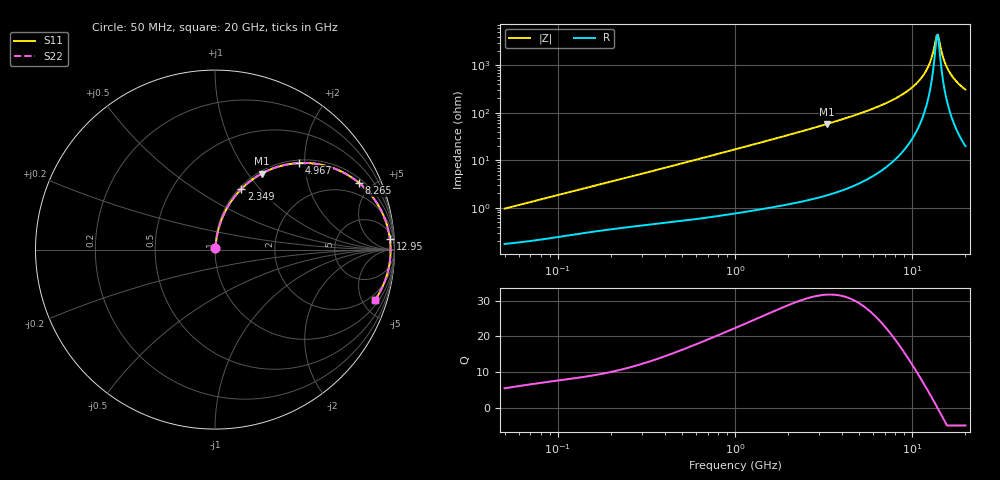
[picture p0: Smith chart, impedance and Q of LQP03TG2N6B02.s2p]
!Murata Part Number: LQP03TG2N6B02
!These Parameters are Measured in Series Mode Connection
!  o--[Z]--o
!Port1  Port2
!  o-------o
!Freq. Start=50[MHz] Stop=20[GHz], 401[Steps]
# Hz S RI R 50
!Freq.(Hz) S11(Real) S11(Imag) S21(Real) S21(Imag) S12(Real) S12(Imag) S22(Real) S22(Imag)
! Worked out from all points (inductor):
!   401 points, 50 MHz to 20 GHz, reference 50 ohm
!   read as one part in series: L = 2.98 nH near 51.52 MHz
!   highest Q = 31.7 at 3.314 GHz (marker M1), where L = 2.79 nH
!   self-resonance near 13.75 GHz
!   S11 on the Smith chart (normalised r, x): 50 MHz: 1.00, +0.02; 2.349 GHz: 1.03, +0.80; 4.967 GHz: 1.06, +1.88; 8.265 GHz: 1.23, +4.21; 12.95 GHz: 12, +29; 20 GHz: 1.40, -6.13
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5e7  0.00182 0.0094  0.9982 -0.0094  0.9982 -0.0094  0.00182 0.0094
1.364002e8  0.00348 0.0245  0.9965 -0.0245  0.9965 -0.0245  0.00348 0.0245
3.721004e8  0.00867 0.0634  0.9913 -0.0634  0.9913 -0.0634  0.00867 0.0634
1e9  0.0348 0.1621  0.9652 -0.1621  0.9652 -0.1621  0.0348 0.1621
2.348516e9  0.147 0.3379  0.853 -0.3379  0.853 -0.3379  0.147 0.3379
2.728004e9  0.189 0.3758  0.811 -0.3758  0.811 -0.3758  0.189 0.3758
3.314454e9  0.2595 0.4229  0.7405 -0.4229  0.7405 -0.4229  0.2595 0.4229
4.966507e9  0.4702 0.4824  0.5298 -0.4824  0.5298 -0.4824  0.4702 0.4824
7.442007e9  0.7376 0.417  0.2624 -0.417  0.2624 -0.417  0.7376 0.417
8.264682e9  0.8032 0.3711  0.1968 -0.3711  0.1968 -0.3711  0.8032 0.3711
9.745021e9  0.8913 0.2752  0.1087 -0.2752  0.1087 -0.2752  0.8913 0.2752
1.098561e10  0.9387 0.1899  0.0613 -0.1899  0.0613 -0.1899  0.9387 0.1899
1.201863e10  0.9628 0.1197  0.0372 -0.1197  0.0372 -0.1197  0.9628 0.1197
1.257102e10  0.9707 0.0832  0.0293 -0.0832  0.0293 -0.0832  0.9707 0.0832
1.295331e10  0.9745 0.0585  0.0255 -0.0585  0.0255 -0.0585  0.9745 0.0585
1.354865e10  0.9778 0.0212  0.0222 -0.0212  0.0222 -0.0212  0.9778 0.0212
1.396067e10  0.9783 -0.00382  0.0217 0.00382  0.0217 0.00382  0.9783 -0.00382
1.417136e10  0.9781 -0.0163  0.0219 0.0163  0.0219 0.0163  0.9781 -0.0163
1.527346e10  0.9723 -0.0786  0.0277 0.0786  0.0277 0.0786  0.9723 -0.0786
1.621653e10  0.962 -0.1274  0.038 0.1274  0.038 0.1274  0.962 -0.1274
1.774144e10  0.9375 -0.1977  0.0625 0.1977  0.0625 0.1977  0.9375 -0.1977
2e10  0.8893 -0.283  0.1107 0.283  0.1107 0.283  0.8893 -0.283
